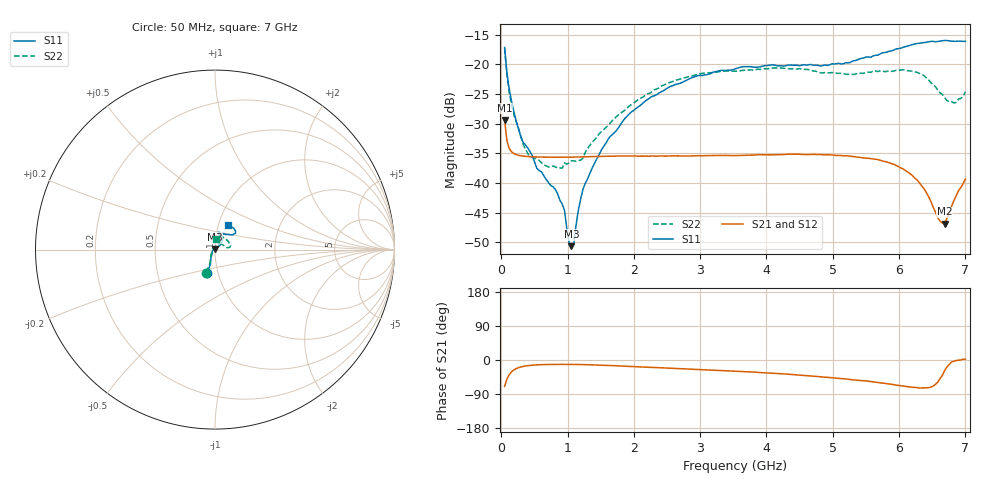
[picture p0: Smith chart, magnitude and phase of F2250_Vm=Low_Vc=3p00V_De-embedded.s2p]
! Integrated Device Technology
! Corporate Headquarters
! 6024 Silver Creek Valley Road
! San Jose, CA 95138  USA
! Phone:  1-408-284-8200
! Toll Free:  1-800-223-1366
! Webpage:  http://www.idt.com/
! Timing and RF Division
! 515 Groton Road, Suite 102
! Westford, MA 01886-6024
! Device:  F2250
! Description: Voltage Variable RF Attenuator
! Frequency:  50.0 -  6000.00 MHz
! Package:  3x3 mm Thin QFN Plastic Package: 16 pin
! Ports:  2 RF, 3 DC
!  Pin  1  = GND
!  Pin  2  = NC
!  Pin  3  = RF1  = Port 1
!  Pin  4  = NC
!  Pin  5  = GND
!  Pin  6  = GND
!  Pin  7  = GND
!  Pin  8  = GND
!  Pin  9  = NC
!  Pin 10  = RF2  = Port 2
!  Pin 11  = NC
!  Pin 12  = GND
!  Pin 13  = GND
!  Pin 14  = VCNTRL
!  Pin 15  = VDD
!  Pin 16  = VMODE
! Vcntrl:  3.000 Volts
! Vmode:  +0.000 Volts
! Vdd:  +3.30  Volts
! Current:  1.175 mA
! Data:  The device was measured on a the F2250 evaluation board which has
!  individual transmission lines to the RF pins.  Data was collected
!  using a calibrated network analyzer.  The evaluation board was
!  de-embedded using a TRL calibration technique.
!  The reference plane is the edge of the package pin.
! Misc:  SN 10
!  Action Tracker AT0258
! Date Measured:  2014-11-26
! Date:  2015-10-15  MJV
! Note:
!  Integrated Device Technology supplies this data as a sample of measured
!  data at the package pin for this product.  Your particular data for this
!  product may vary.
!  Data was taken at 25 degrees C.
!  Integrated Device Technology reserves the right to change this data at anytime.
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# GHz S dB R 50
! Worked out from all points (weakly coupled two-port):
!   201 points, 50 MHz to 7 GHz, reference 50 ohm
!   highest |S21| = -29.41 dB at 50 MHz (marker M1); lowest = -46.9 dB at 6.687 GHz (marker M2)
!   lowest |S11| = -50.7 dB at 1.058 GHz (marker M3), VSWR 1.01, Z = 49.8 + j0.245 ohm
!   |S11| at or under -10 dB: start of sweep to end of sweep
!   |S22| runs from -37.5 to -17.3 dB; largest |S21 - S12| = 6.3e-05
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0.05  -17.18 -108.6  -29.41 -69.8  -29.41 -69.8  -17.28 -111.0
0.08475  -21.44 -107.5  -32.92 -50.4  -32.92 -50.3  -21.74 -110.2
0.15425  -26.23 -116.6  -34.76 -31.1  -34.76 -31.2  -26.81 -122.5
0.29325  -32.21 -127.8  -35.43 -18.5  -35.43 -18.5  -32.08 -137.3
0.3975  -34.08 -141.8  -35.56 -15.0  -35.56 -15.0  -35.04 -160.4
0.5365  -37.57 -155.7  -35.64 -12.8  -35.63 -12.9  -36.04 178.0
0.91875  -43.58 158.0  -35.69 -11.5  -35.68 -11.5  -37.53 133.5
0.9535  -44.62 169.9  -35.68 -11.5  -35.68 -11.5  -36.65 131.0
1.023  -50.09 143.7  -35.67 -11.6  -35.67 -11.6  -36.64 116.0
1.05775  -50.68 123.0  -35.67 -11.6  -35.67 -11.6  -36.28 110.7
1.0925  -50.41 90.5  -35.66 -11.7  -35.65 -11.7  -36.30 106.4
1.162  -44.62 57.1  -35.64 -11.9  -35.64 -11.9  -36.21 95.4
1.2315  -41.10 44.3  -35.61 -12.1  -35.61 -12.1  -35.81 85.8
1.6485  -32.11 41.9  -35.52 -14.6  -35.51 -14.6  -29.87 64.5
2.37825  -24.87 47.3  -35.48 -20.3  -35.48 -20.3  -23.99 56.7
3.525  -20.79 72.4  -35.40 -29.5  -35.40 -29.5  -21.19 74.7
4.7065  -20.17 72.3  -35.19 -42.6  -35.19 -42.6  -21.14 72.2
5.85325  -17.81 40.5  -36.64 -63.4  -36.63 -63.5  -21.15 23.1
6.27025  -16.51 40.0  -39.49 -72.8  -39.51 -72.9  -21.37 9.7
6.68725  -15.99 48.7  -46.88 -27.6  -46.86 -27.3  -25.63 28.7
6.861  -16.14 55.1  -42.20 -1.4  -42.14 -1.4  -26.45 57.9
7  -16.13 63.2  -39.37 1.8  -39.34 1.7  -24.64 83.1
